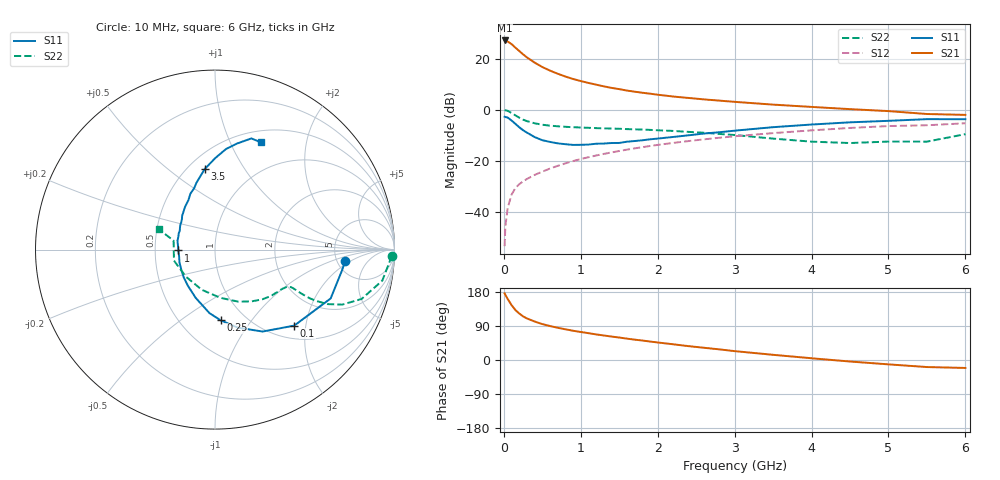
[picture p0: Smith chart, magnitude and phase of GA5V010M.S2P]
! Infineon Technologies  Discrete & RF Semiconductors
! BF775
! Si NPN RF Bipolar Junction Transistor in SOT23
! VCE = 5 V  IC = 10 mA
! Common Emitter S-Parameters:  May  1996
# GHz  S  MA  R  50
!  f  S11  S21  S12  S22
! GHz  MAG  ANG  MAG  ANG  MAG  ANG  MAG  ANG
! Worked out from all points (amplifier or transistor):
!   36 points, 10 MHz to 6 GHz, reference 50 ohm
!   highest |S21| = 27.2 dB at 10 MHz (marker M1)
!   |S21| within 3 dB of that: start of sweep to 157 MHz
!   unconditionally stable (mu >= 1): 591.9 MHz to 3.031 GHz
!   at 250 MHz: K = 0.68, MSG = 24.9 dB, |S12| = -28.1 dB
!   at 1.4 GHz: K = 1.10, MAG = 10.7 dB, |S12| = -16.8 dB
!   at 6 GHz: K = 0.93, MSG = 1.6 dB, |S12| = -5.3 dB
!   S11 on the Smith chart (normalised r, x): 10 MHz: 5.93, -1.57; 100 MHz: 1.27, -1.72; 250 MHz: 0.77, -0.72; 1 GHz: 0.66, -0.01; 3.5 GHz: 0.60, +0.68; 6 GHz: 0.63, +1.31
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0.01  0.7281 -4.9  22.78 175.8  0.0021 88.9  0.985 -2.0
0.02  0.7167 -9.5  22.33 171.8  0.0052 83.5  0.973 -4.4
0.05  0.6994 -22.9  21.68 161.0  0.0118 79.6  0.9481 -10.5
0.1  0.6119 -43.8  19.33 144.9  0.0215 70.9  0.862 -18.6
0.15  0.5277 -59.9  16.47 132.0  0.0289 66.0  0.772 -23.4
0.2  0.4525 -73.8  14.17 122.6  0.0345 64.2  0.6977 -25.8
0.25  0.3949 -85.5  12.17 115.2  0.0392 62.3  0.6375 -26.8
0.3  0.3551 -95.0  10.6 109.7  0.0437 62.5  0.5957 -27.2
0.4  0.29 -111.7  8.384 101.6  0.0525 62.9  0.5415 -27.0
0.5  0.252 -126.8  6.858 94.8  0.0608 63.8  0.5064 -26.6
0.6  0.233 -138.4  5.835 89.6  0.07 64.6  0.4856 -26.3
0.7  0.2182 -149.5  5.071 85.1  0.079 65.4  0.4721 -26.3
0.8  0.2103 -160.3  4.467 81.0  0.0884 65.2  0.461 -26.7
1  0.2043 -178.6  3.643 73.9  0.1074 65.1  0.4468 -28.0
1.1  0.2067 174.9  3.343 70.8  0.1167 64.8  0.4407 -29.2
1.3  0.2163 161.1  2.863 64.7  0.1357 63.9  0.4299 -31.3
1.6  0.2353 145.6  2.372 56.4  0.1643 61.8  0.4154 -35.6
2.2  0.2913 124.9  1.811 41.5  0.2225 56.5  0.3827 -46.3
3.5  0.4532 97.2  1.256 13.7  0.3467 41.8  0.2704 -83.5
4.5  0.5642 83.7  1.024 -4.0  0.4377 29.1  0.2214 -136.9
5.5  0.6517 71.9  0.822 -18.6  0.4945 14.1  0.236 167.8
6  0.6498 66.8  0.79 -21.0  0.5409 10.1  0.3309 160.2
